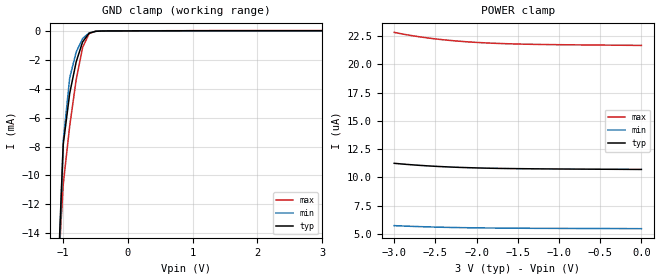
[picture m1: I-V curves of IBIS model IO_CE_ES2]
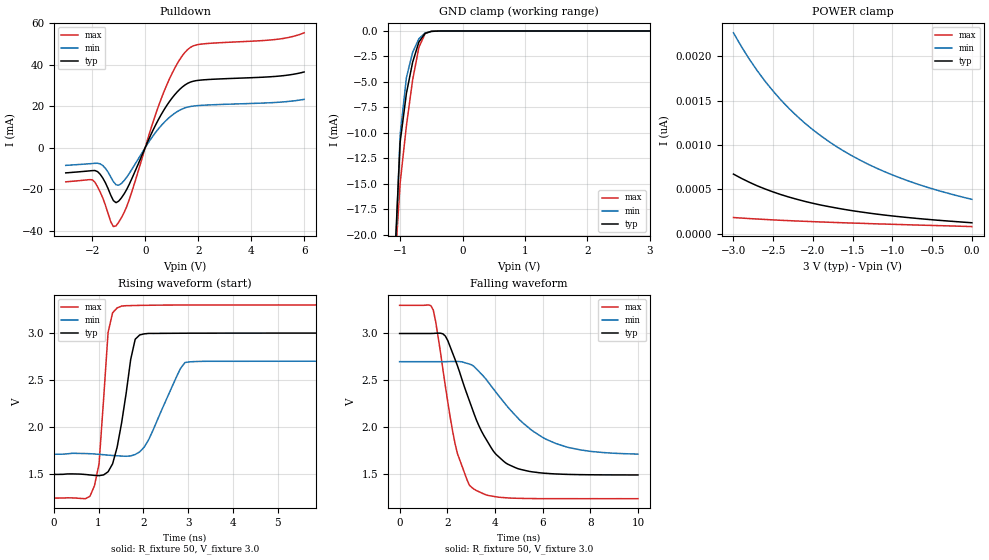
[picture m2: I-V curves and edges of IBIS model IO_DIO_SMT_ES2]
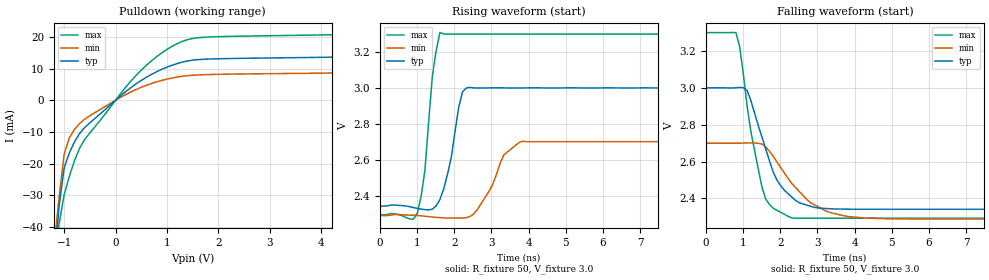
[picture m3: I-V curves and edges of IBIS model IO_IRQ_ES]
[IBIS Ver]   3.2
[Comment Char]   |_char
[File name]   r8900sa_3.ibs
[File Rev]   1.0
[Date]   2016/03/15
[Source]   This file orginated at SEIKO EPSON Corp.
[Notes]
[Disclaimer]
This information is for modeling purposes only, and is not guaranteed.
Property of SEIKO EPSON Corp.,
unauthorized reproduction and/or distribution is strictly prohibited.
[Copyright]
Copyright 2016, SEIKO EPSON Corp.
[Component]   r8900sa_3
Si_location Pin
Timing_location Pin
[Manufacturer]   SEIKO EPSON Corp.
[Package]
R_pkg   3.00m   NA   NA
L_pkg   3.70nH   NA   NA
C_pkg   0.70pF   NA   NA
[Pin] signal_name   model_name
1   CE   IO_CE_ES2
2   SCL   IO_INSPD2_ES2
3   FOUT   IO_OUT_ES
|4   N.C.
|5   VBAT   POWER2
6   VDD   POWER
7   FOE   IO_INSPD3_ES2
|8   N.C.
|9   N.C.
10   _INT   IO_IRQ_ES
11   VSS   POWER
|12   T2   TEST2
13   SDA   IO_DIO_SMT_ES2
| Models and submodels in the file (6): IO_CE_ES2 (Input), IO_DIO_SMT_ES2 (I/O_open_drain), IO_IRQ_ES (Open_drain), IO_INSPD3_ES2 (Input), IO_OUT_ES (3-state), IO_INSPD2_ES2 (Input)
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|14   N.C.
[Model]   IO_CE_ES2
Model_type Input
Enable Active-Low
Polarity Non-Inverting
Vinh=2.4
Vinl=0.6
C_comp   2.5p   2p   3p
[Temperature Range] 25   85   -40
[Voltage Range]   3.0   2.7   3.3
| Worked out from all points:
|   GND clamp passes 1 mA (typ) near -0.72 V on its own axis
[GND Clamp]
-3V       -391.4mA   -327.7mA   -491.9mA
-1.1V     -19.19mA   -20.81mA   -18.41mA
-1V       -7.867mA   -7.623mA   -10.62mA
-900mV    -4.321mA   -3.247mA   -6.585mA
-800mV    -2.143mA   -1.467mA   -3.376mA
-700mV    -757.1uA   -529.2uA   -1.136mA
-600mV    -163.2uA   -135.5uA   -183.6uA
-500mV    -29.95uA   -29.59uA   -27.27uA
-400mV    -8.459uA   -7.518uA   -10.52uA
3V        10.7uA     5.475uA    21.65uA
[POWER Clamp]
-3V       11.25uA    5.735uA    22.83uA
-2.8V     11.12uA    5.675uA    22.56uA
-2.7V     11.07uA    5.649uA    22.44uA
-2.5V     10.98uA    5.607uA    22.25uA
-2.4V     10.95uA    5.589uA    22.17uA
-2.2V     10.89uA    5.56uA     22.04uA
-2.1V     10.86uA    5.548uA    21.99uA
-1.9V     10.82uA    5.53uA     21.9uA
-1.6V     10.78uA    5.511uA    21.82uA
-1.3V     10.76uA    5.499uA    21.77uA
-900mV    10.74uA    5.488uA    21.73uA
0V        10.7uA     5.467uA    21.67uA
[Model]   IO_DIO_SMT_ES2
Model_type I/O_open_drain
Enable Active-High
Polarity Non-Inverting
Vinh=2.4
Vinl=0.6
Vref=3.3
Vmeas=1.5
Rref=5000
C_comp   2.5p   2p   3p
[Temperature Range] 25   85   -40
[Voltage Range]   3.0   2.7   3.3
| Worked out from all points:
|   slope of the pulldown table from 0 to 0.45 V, typ, clamps not added: 36.5 ohm
|   GND clamp passes 1 mA (typ) near -0.69 V on its own axis
|   falling waveform, R_fixture 50, V_fixture 3.0: 20-80 % time 1.45ns typ, 2.23ns min, 863ps max; typ from 3 V to 1.49 V
|   rising waveform, R_fixture 50, V_fixture 3.0: 20-80 % time 293ps typ, 550ps min, 178ps max; typ from 1.49 V to 3 V
[Pulldown]
-3V       -12.19mA   -8.567mA   -16.5mA
-2V       -11.1mA    -7.676mA   -15.51mA
-1.6V     -14.7mA    -8.655mA   -24.32mA
-1.3V     -22.98mA   -14.16mA   -35.77mA
-1.1V     -26.54mA   -17.92mA   -37.73mA
-600mV    -17.64mA   -12.42mA   -25.02mA
300mV     8.527mA    5.742mA    12.5mA
700mV     18.02mA    11.94mA    26.7mA
1.2V      26.75mA    17.29mA    40.29mA
1.6V      30.98mA    19.54mA    47.25mA
2.1V      32.57mA    20.37mA    49.89mA
6V        36.47mA    23.28mA    55.36mA
[GND Clamp]
-3V       -509mA     -424.1mA   -637.2mA
-1.1V     -24.22mA   -25.63mA   -24.62mA
-1V       -10.89mA   -10.16mA   -14.91mA
-900mV    -6.131mA   -4.569mA   -9.309mA
-800mV    -3.058mA   -2.097mA   -4.786mA
-700mV    -1.078mA   -757.4uA   -1.604mA
-600mV    -224.6uA   -189.6uA   -244.1uA
-500mV    -33.81uA   -37.1uA    -22.82uA
-400mV    -4.624uA   -6.222uA   -2.07uA
3V        124.3pA    456.2pA    73.5pA
[POWER Clamp]
-3V       671.8pA    2.262nA    182.9pA
-2.8V     580pA      1.965nA    171.3pA
-2.6V     503.6pA    1.715nA    161.1pA
-2.5V     470.8pA    1.605nA    156.5pA
-2.4V     440.3pA    1.503nA    151.7pA
-2.2V     388pA      1.324nA    143.8pA
-2V       343.1pA    1.17nA     136.8pA
-1.8V     306pA      1.039nA    129.9pA
-1.4V     246.3pA    825.9pA    118.2pA
-1V       200.8pA    662.6pA    106.6pA
-600mV    165.5pA    534.6pA    96.35pA
0V        124.3pA    388.2pA    81.06pA
[Falling Waveform]
R_fixture=50
V_fixture=3.0
V_fixture_min=2.7
V_fixture_max=3.3
0s        3V         2.7V       3.3V
1.414ns   3.001V     2.7V       3.249V
1.919ns   2.973V     2.7V       2.44V
2.323ns   2.726V     2.702V     1.831V
2.828ns   2.354V     2.682V     1.442V
3.03ns    2.211V     2.665V     1.36V
3.939ns   1.745V     2.408V     1.265V
4.949ns   1.562V     2.103V     1.245V
6.97ns    1.5V       1.795V     1.241V
10ns      1.494V     1.715V     1.241V
[Rising Waveform]
R_fixture=50
V_fixture=3.0
V_fixture_min=2.7
V_fixture_max=3.3
0s        1.493V     1.708V     1.241V
707.1ps   1.492V     1.715V     1.234V
909.1ps   1.483V     1.711V     1.374V
1.01ns    1.48V      1.707V     1.605V
1.212ns   1.521V     1.699V     3.007V
1.414ns   1.782V     1.692V     3.268V
1.717ns   2.718V     1.691V     3.293V
1.919ns   2.98V      1.734V     3.295V
2.929ns   2.998V     2.685V     3.299V
10ns      3V         2.7V       3.3V
[Ramp]
R_load=50
dV/dt_r   9.040E-1/2.903E-10   5.949E-1/5.488E-10   1.235E+0/1.711E-10
dV/dt_f   9.039E-1/1.450E-9   5.907E-1/2.229E-9   1.235E+0/8.622E-10
|[End   IO_DIO_SMT_ES2
[Model]   IO_IRQ_ES
Model_type Open_drain
Enable Active-Low
Polarity Non-Inverting
Vref=3.3
Vmeas=1.5
Rref=5000
C_comp   2.5p   2p   3p
[Temperature Range] 25   85   -40
[Voltage Range]   3.0   2.7   3.3
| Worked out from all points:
|   slope of the pulldown table from 0 to 0.45 V, typ, clamps not added: 78.7 ohm
|   falling waveform, R_fixture 50, V_fixture 3.0: 20-80 % time 699ps typ, 1.03ns min, 484ps max; typ from 3 V to 2.34 V
|   rising waveform, R_fixture 50, V_fixture 3.0: 20-80 % time 342ps typ, 543ps min, 256ps max; typ from 2.34 V to 3 V
[Pulldown]
-3V       -460.3mA   -383.6mA   -577.8mA
-1.2V     -53.34mA   -46.96mA   -63.7mA
-1.1V     -33.78mA   -31.03mA   -39.25mA
-1V       -21.42mA   -17.13mA   -29.89mA
-900mV    -16.66mA   -11.93mA   -24.12mA
-700mV    -10.51mA   -7.336mA   -15.14mA
400mV     5.176mA    3.38mA     7.841mA
900mV     9.765mA    6.259mA    14.95mA
1.3V      12.03mA    7.562mA    18.56mA
1.8V      12.97mA    8.09mA     19.92mA
4.8V      13.77mA    8.724mA    20.93mA
6V        14.9mA     9.477mA    22.76mA
[Falling Waveform]
R_fixture=50
V_fixture=3.0
V_fixture_min=2.7
V_fixture_max=3.3
0s        3V         2.7V       3.3V
808.1ps   3V         2.7V       3.3V
909.1ps   3.003V     2.7V       3.223V
1.111ns   2.985V     2.701V     2.898V
1.515ns   2.728V     2.694V     2.456V
1.818ns   2.54V      2.626V     2.346V
2.222ns   2.424V     2.505V     2.302V
2.828ns   2.357V     2.375V     2.292V
3.838ns   2.341V     2.301V     2.292V
10ns      2.341V     2.288V     2.292V
[Rising Waveform]
R_fixture=50
V_fixture=3.0
V_fixture_min=2.7
V_fixture_max=3.3
0s        2.341V     2.288V     2.292V
1.01ns    2.328V     2.289V     2.302V
1.212ns   2.321V     2.284V     2.54V
1.414ns   2.324V     2.28V      3.069V
1.616ns   2.378V     2.277V     3.309V
1.919ns   2.61V      2.274V     3.3V
2.121ns   2.891V     2.275V     3.3V
2.323ns   2.999V     2.276V     3.3V
3.838ns   3V         2.703V     3.3V
10ns      3V         2.7V       3.3V
[Ramp]
R_load=50
dV/dt_r   3.955E-1/3.366E-10   2.473E-1/5.230E-10   6.046E-1/2.462E-10
dV/dt_f   3.955E-1/6.961E-10   2.472E-1/1.026E-9   6.046E-1/4.788E-10
|[End   IO_IRQ_ES
